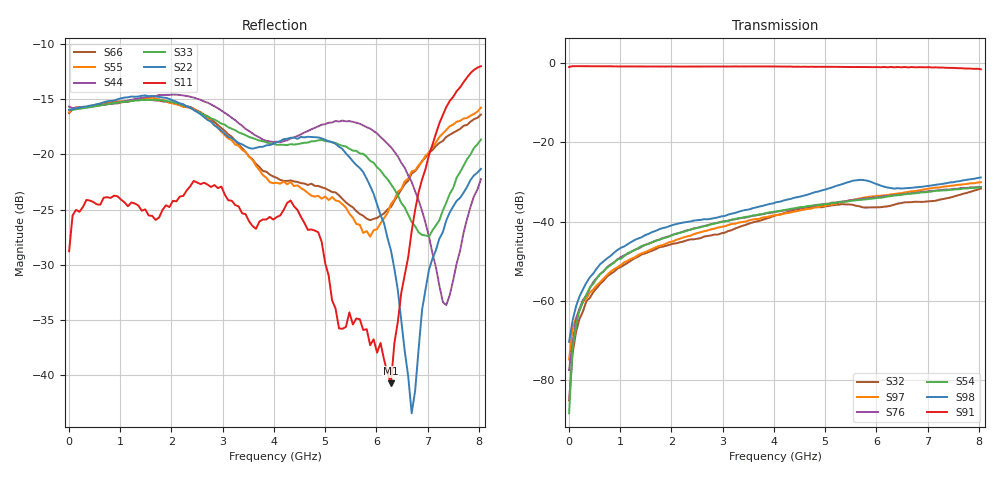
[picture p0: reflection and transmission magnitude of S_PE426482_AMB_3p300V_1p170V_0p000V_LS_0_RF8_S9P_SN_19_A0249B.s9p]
! Device ID: PE426482
! File Path: z:\PE426482\Final Char Data\room\AMB\3p300\LS_0_RF8\PE426482_AMB_3p300V_1p170V_0p000V_LS_0_RF8_S9P_SN_19_A0249B.s9p
! Serial: 19
! Lot: A0249B
! Temp: AMB
! VDD: 3.300
! VSS: 0.000
! Control_Hi: 1.170
! Control_Lo: 0.000
! Logic State: LS_0_RF8
! Port 1:
! Port 2:
! Port 3:
! Port 4:
! Port 5:
! Port 6:
! Port 7:
! Port 8:
! Port 9:
! ThroughPath:1-9
! IDD: 0.0001099221
! ISS/IDD2: -1.67e-008
! IDMM3/IDD3: -1.926e-007
! Comment:
#  Hz  S  RI  R  50
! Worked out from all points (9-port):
!   120 points, 10 MHz to 8.037 GHz, reference 50 ohm
!   strongest paths, dB at 10 MHz, 2.034 GHz, 4.057 GHz, 6.08 GHz, 8.037 GHz:
!     S91: -0.9, -0.8, -0.8, -1.0, -1.5
!     S98: -70.3, -40.8, -35.0, -30.9, -28.8
!     S54: -88.3, -43.3, -37.4, -33.9, -31.3
!     S76: -77.4, -43.3, -37.5, -33.7, -31.2
!     S97: -74.8, -45.0, -38.3, -33.4, -30.0
!     S32: -85.1, -45.5, -38.3, -36.3, -31.6
!   lowest |S11| = -40.7 dB at 6.283 GHz (marker M1), VSWR 1.02, Z = 50.2 + j0.905 ohm
!   |S11| at or under -10 dB: start of sweep to end of sweep
